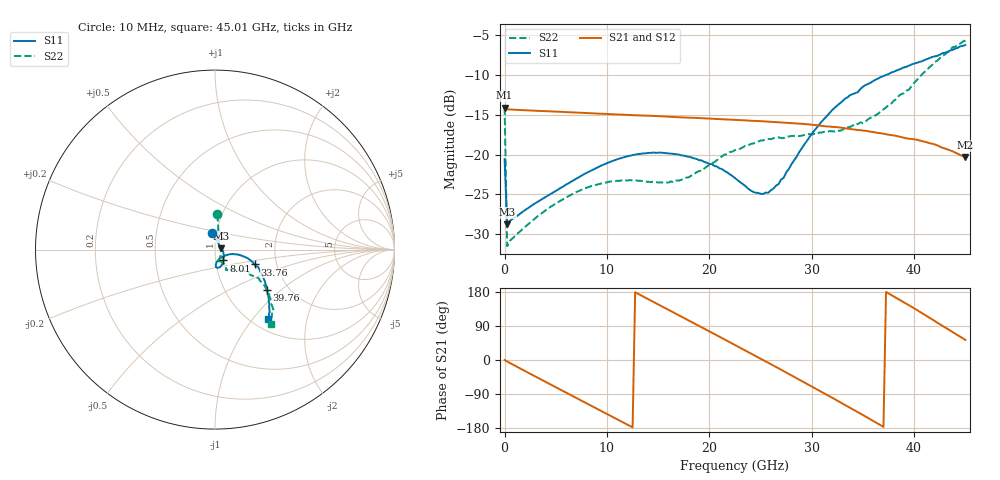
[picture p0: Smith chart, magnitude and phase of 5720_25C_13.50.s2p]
! Device:  ADRF5720
! Description: 0.5dB LSB GaAs MMIC 6-bit Digital Attenuator
! Frequency:  0.000009 -  40 GHz
! Ports:
!	RF1	= Port 1
!	RF2	= Port 2
! Vdd:  3.3 Volt
! Vss:  -3.3 Volt
! Control:  0/3.3 Volt
! State:  13.50 dB attenuation
! Data:  The device was measured using G-S-G Probes on a matrix board.
!  Data was collected using an calibrated 4 port network analyzer.
!  The reference plane for this measurement is at the launchers.
! Note:  Analog Devices supplies this data as a sample of measured data
!  for this product.  Your particular data for this product may vary.
!  Data was taken at 25 degrees C.
!  Analog Devices reserves the right to change this data at anytime.
# GHZ S DB R 45.0
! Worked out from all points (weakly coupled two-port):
!   181 points, 10 MHz to 45.01 GHz, reference 45 ohm
!   highest |S21| = -14.14 dB at 10 MHz (marker M1); lowest = -20.4 dB at 45.01 GHz (marker M2)
!   lowest |S11| = -28.8 dB at 260 MHz (marker M3), VSWR 1.08, Z = 48.3 + j0.796 ohm
!   |S11| at or under -10 dB: start of sweep to 37.3 GHz
!   |S22| runs from -31.5 to -5.7 dB; largest |S21 - S12| = 0.00027
!   S11 on the Smith chart (normalised r, x): 10 MHz: 0.95, +0.18; 8.01 GHz: 1.09, -0.13; 33.76 GHz: 1.54, -0.27; 39.76 GHz: 1.56, -0.81; 45.01 GHz: 1.18, -1.20
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0.01  -20.57 100.2  -14.14 -0.0  -14.14 -0.0  -14.12 86.1
0.26  -28.76 13.0  -14.33 -4.0  -14.33 -4.0  -31.49 16.5
1.26  -27.68 -2.8  -14.39 -18.5  -14.40 -18.5  -29.92 -8.5
4.26  -25.13 -29.9  -14.57 -61.3  -14.57 -61.2  -26.77 -46.7
7.76  -22.47 -50.9  -14.78 -110.7  -14.78 -110.7  -24.29 -69.3
8.01  -22.30 -52.3  -14.79 -114.3  -14.79 -114.3  -24.15 -70.4
11.76  -20.30 -69.2  -15.01 -167.2  -15.02 -167.1  -23.24 -80.9
15.26  -19.76 -81.1  -15.20 143.2  -15.20 143.2  -23.49 -78.0
16.51  -19.92 -84.0  -15.29 125.4  -15.30 125.4  -23.47 -72.7
19.01  -20.71 -87.3  -15.43 89.8  -15.43 89.8  -22.07 -61.4
22.76  -23.22 -81.5  -15.67 36.1  -15.67 36.1  -19.38 -57.7
24.26  -24.67 -68.3  -15.77 14.5  -15.78 14.5  -18.62 -58.8
25.76  -24.80 -45.3  -15.86 -7.3  -15.87 -7.2  -18.05 -60.2
27.26  -22.92 -24.4  -15.98 -29.3  -15.98 -29.3  -17.94 -60.0
30.26  -16.99 -12.1  -16.29 -73.7  -16.30 -73.7  -17.40 -57.9
33.76  -12.54 -20.5  -16.79 -126.3  -16.79 -126.3  -16.52 -48.2
35.26  -11.28 -24.2  -17.02 -149.2  -17.03 -149.2  -15.87 -43.9
37.76  -9.72 -32.2  -17.55 171.9  -17.55 172.0  -13.62 -35.4
39.76  -8.70 -38.0  -18.04 140.4  -18.04 140.5  -11.40 -33.8
42.26  -7.62 -43.9  -18.85 98.5  -18.85 98.6  -8.22 -39.3
43.76  -6.88 -48.1  -19.59 73.7  -19.59 73.7  -6.51 -46.2
45.01  -6.26 -52.5  -20.35 53.1  -20.35 53.1  -5.69 -52.7
